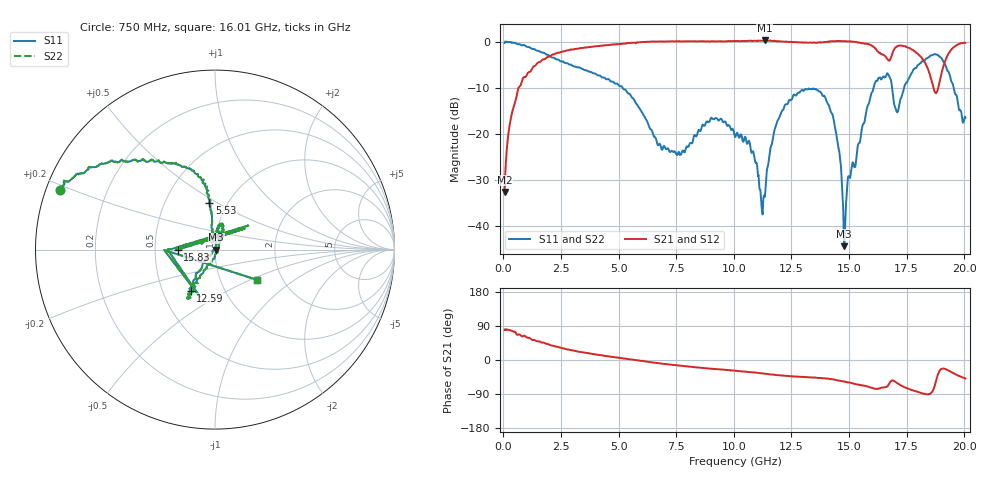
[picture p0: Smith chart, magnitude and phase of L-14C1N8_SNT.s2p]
#	mhz	s	ma	r	50
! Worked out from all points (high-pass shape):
!   1001 points, 50 MHz to 20.05 GHz, reference 50 ohm
!   highest |S21| = 0.30 dB at 11.35 GHz (marker M1); lowest = -32.6 dB at 50 MHz (marker M2)
!   |S21| within 3 dB of the highest: 2.182 GHz to 16.43 GHz (14.25 GHz wide, 153 % of centre); 16.87 GHz to 18.01 GHz (1.138 GHz wide, 6.53 % of centre)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
!   lowest |S11| = -44.3 dB at 14.79 GHz (marker M3), VSWR 1.01, Z = 50.6 + j0.0164 ohm
!   |S11| at or under -10 dB: 5.179 GHz to 16.06 GHz (10.88 GHz wide, 102 % of centre); 16.87 GHz to 17.39 GHz (516.1 MHz wide, 3.01 % of centre); 19.54 GHz to end of sweep
!   |S22| runs from -44.3 to 0.1 dB; largest |S21 - S12| = 0
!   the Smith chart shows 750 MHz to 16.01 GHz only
!   S11 on the Smith chart (normalised r, x): 750 MHz: 0.04, +0.19; 5.53 GHz: 0.82, +0.46; 12.59 GHz: 0.69, -0.34; 15.83 GHz: 0.66, -0.00; 16.01 GHz: 1.49, -0.55
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50  0.9732 178.0  0.02354 79.5  0.02354 79.5  0.9732 178.0
290  0.9907 172.0  0.1341 78.2  0.1341 78.2  0.9907 172.0
750  0.925 159.0  0.3396 65.0  0.3396 65.0  0.925 159.0
3390  0.5126 113.0  0.8582 20.7  0.8582 20.7  0.5126 113.0
5530  0.261 97.0  0.9732 1.5  0.9732 1.5  0.261 97.0
6730  0.07638 91.1  1.009 -8.6  1.009 -8.6  0.07638 91.1
9110  0.1453 75.7  1.015 -23.2  1.015 -23.2  0.1453 75.7
10050  0.09302 81.5  1.024 -28.2  1.024 -28.2  0.09302 81.5
11350  0.02094 -66.9  1.036 -36.2  1.036 -36.2  0.02094 -66.9
11830  0.1239 -116.4  1.016 -39.5  1.016 -39.5  0.1239 -116.4
12590  0.266 -120.7  0.9959 -43.3  0.9959 -43.3  0.266 -120.7
13390  0.3078 -119.7  0.9794 -46.2  0.9794 -46.2  0.3078 -119.7
14310  0.1524 -126.5  1.017 -51.3  1.017 -51.3  0.1524 -126.5
14790  0.0061 1.5  1.015 -56.8  1.015 -56.8  0.0061 1.5
15830  0.2074 -179.9  0.949 -70.6  0.949 -70.6  0.2074 -179.9
16010  0.2874 -35.8  0.9021 -74.0  0.9021 -74.0  0.2874 -35.8
16730  0.4291 148.3  0.627 -63.8  0.627 -63.8  0.4291 148.3
17090  0.172 174.6  0.8932 -61.1  0.8932 -61.1  0.172 174.6
18230  0.6185 -172.3  0.6345 -88.6  0.6345 -88.6  0.6185 -172.3
18830  0.7227 137.1  0.2927 -43.7  0.2927 -43.7  0.7227 137.1
19390  0.4173 96.4  0.7941 -30.0  0.7941 -30.0  0.4173 96.4
20050  0.1503 133.0  0.9754 -48.8  0.9754 -48.8  0.1503 133.0
